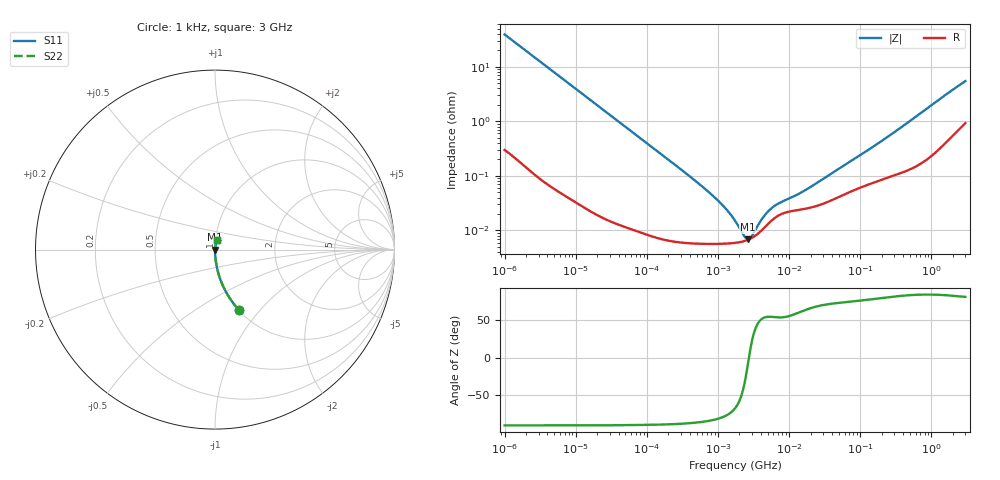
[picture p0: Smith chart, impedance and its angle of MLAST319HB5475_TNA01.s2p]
! MLAST319HB5475_TNA01  S-PARAMETER MODEL  ( Standard Model )
! Model Generated by TAIYO YUDEN Corporation (http://www.ty-top.com)
! Version 1.0
! TAIYO YUDEN Control No. 220601
! Copyright(c) 2009 TAIYO YUDEN CO.,LTD. All Rights Reserved.
! Product Description (link to TY-COMPAS)
! https://ds.yuden.co.jp/TYCOMPAS/or/detail?pn=MLAST319HB5475KTNA01&u=M
! Products Name : Multilayer Ceramic Capacitors
! Characteristics :
!  Capacitance : 4.7 [uF] , Rated Voltage : 25 [V] , TCC : X5R
!  Case Size : 3.2 x 1.6 / 0.126 x 0.063 [mm/inch] , Thickness : 0.85 / 0.033 [mm/inch]
!  (Conditions: Temperature = 25 [degC] , DC Bias Voltage = 0 [V])
! External Node Assignments :
!  1  o---| |---o  2
! GND o---------o GND
! Frequency Range : 1kHz  -  3GHz  [ 401 STEP ]
# MHZ S RI R 50
! Freq[MHz].  S11 Real  S11 Imag  S21 Real  S21 Imag  S12 Real  S12 Imag  S22 Real  S22 Imag
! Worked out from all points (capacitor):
!   401 points, 1 kHz to 3 GHz, reference 50 ohm
!   read as one part in series: C = 4.09 uF near 1.077 kHz
!   lowest |Z| = 6.82 mohm at 2.61 MHz (marker M1)
!   series resonance near 2.72 MHz, so ESL is about 840 pH
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0.001  0.1333 -0.336  0.8667 0.336  0.8667 0.336  0.1333 -0.336
0.001685  0.0523 -0.2189  0.9477 0.2189  0.9477 0.2189  0.0523 -0.2189
0.00306  0.0169 -0.1255  0.9831 0.1255  0.9831 0.1255  0.0169 -0.1255
0.005768  0.0051 -0.0676  0.9949 0.0676  0.9949 0.0676  0.0051 -0.0676
0.01216  0.00132 -0.0323  0.9987 0.0323  0.9987 0.0323  0.00132 -0.0323
0.147855  7.84e-05 -0.00269  0.9999 0.00269  0.9999 0.00269  7.84e-05 -0.00269
0.43594  5.85e-05 -0.000893  0.9999 0.000893  0.9999 0.000893  5.85e-05 -0.000893
0.821683  5.67e-05 -0.000444  0.9999 0.000444  0.9999 0.000444  5.67e-05 -0.000444
1.238299  5.72e-05 -0.000258  0.9999 0.000258  0.9999 0.000258  5.72e-05 -0.000258
1.732051  5.91e-05 -0.000139  0.9999 0.000139  0.9999 0.000139  5.91e-05 -0.000139
2.087011  6.15e-05 -8.03e-05  0.9999 8.03e-05  0.9999 8.03e-05  6.15e-05 -8.03e-05
2.24859  6.29e-05 -5.75e-05  0.9999 5.75e-05  0.9999 5.75e-05  6.29e-05 -5.75e-05
2.610246  6.71e-05 -1.24e-05  0.9999 1.24e-05  0.9999 1.24e-05  6.71e-05 -1.24e-05
3.14518  7.59e-05 4.38e-05  0.9999 -4.38e-05  0.9999 -4.38e-05  7.59e-05 4.38e-05
3.388684  8.11e-05 6.64e-05  0.9999 -6.64e-05  0.9999 -6.64e-05  8.11e-05 6.64e-05
4.566395  0.000115 0.000154  0.9999 -0.000154  0.9999 -0.000154  0.000115 0.000154
6.153411  0.000165 0.000224  0.9998 -0.000224  0.9998 -0.000224  0.000165 0.000224
13.97519  0.000239 0.000412  0.9998 -0.000412  0.9998 -0.000412  0.000239 0.000412
21.06097  0.000266 0.000595  0.9997 -0.000595  0.9997 -0.000595  0.000266 0.000595
256.0921  0.000974 0.00535  0.999 -0.00535  0.999 -0.00535  0.000974 0.00535
1714.862  0.00549 0.0323  0.9945 -0.0323  0.9945 -0.0323  0.00549 0.0323
3000  0.0119 0.0525  0.9881 -0.0525  0.9881 -0.0525  0.0119 0.0525
